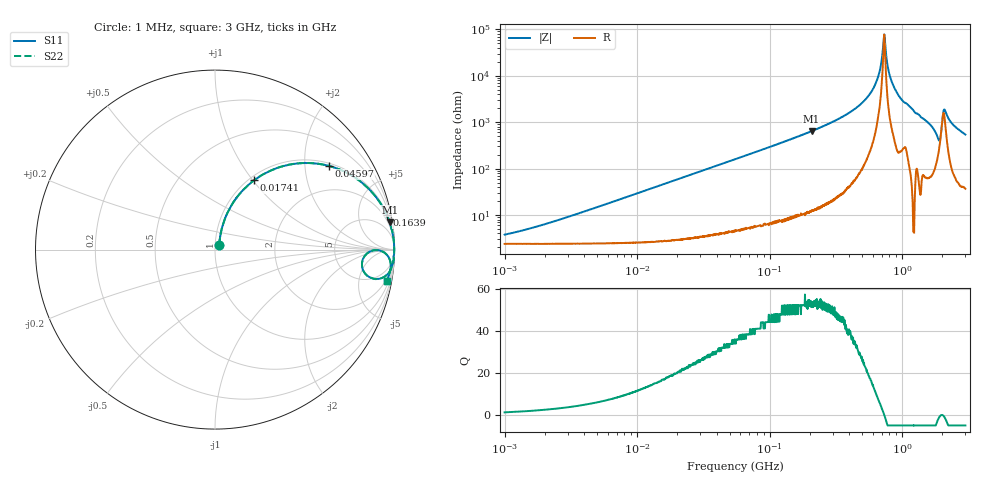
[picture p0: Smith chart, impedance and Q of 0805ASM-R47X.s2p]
!s-Parameter Generated by FASTRON Sdn. Bhd.
!FASTRON P/N : 0805ASM-R47X
!Keysight Technologies: E4991B_MY54100416_A.01.15
!Date: Fri Jun 19 14:52:53 2026
!Version  :Rev00  Fri Jun 19 14:52:53 2026
!Data & Calibration Information:
!Freq  S11  S21  S12  S22
!PortZ  Port1:50+j0  Port2:50+j0
!When reading reference impedance value at option line is always used.
! Remarks : This data is being provided solely for informational purposes.
# Hz S dB R 50
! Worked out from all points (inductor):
!   1601 points, 1 MHz to 3 GHz, reference 50 ohm
!   read as one part in series: L = 465 nH near 2.474 MHz
!   highest Q = 54 at 207.3 MHz (marker M1), where L = 494 nH
!   self-resonance near 731.6 MHz
!   S11 on the Smith chart (normalised r, x): 1 MHz: 1.05, +0.06; 17.41 MHz: 1.06, +1.01; 45.97 MHz: 1.08, +2.67; 163.9 MHz: 1.20, +9.87; 3 GHz: 2, -11
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1000000  -28.70 49.1  -0.21 -1.6  -0.21 -1.6  -28.70 49.1
3804036  -19.10 71.5  -0.26 -6.2  -0.26 -6.2  -19.10 71.5
1.447069e7  -8.39 64.0  -0.91 -22.3  -0.91 -22.3  -8.39 64.0
1.741396e7  -7.07 60.6  -1.19 -26.3  -1.19 -26.3  -7.07 60.6
4.597255e7  -2.06 36.2  -4.57 -52.0  -4.57 -52.0  -2.06 36.2
5.504702e7  -1.55 31.6  -5.62 -56.8  -5.62 -56.8  -1.55 31.6
1.63867e8  -0.21 11.4  -14.00 -77.4  -14.00 -77.4  -0.21 11.4
2.073156e8  -0.13 8.8  -16.30 -80.1  -16.30 -80.1  -0.13 8.8
2.083556e8  -0.13 8.8  -16.30 -80.1  -16.30 -80.1  -0.13 8.8
3.760477e8  -0.04 4.0  -23.20 -84.7  -23.20 -84.7  -0.04 4.0
5.391547e8  -0.02 1.7  -30.40 -85.5  -30.40 -85.5  -0.02 1.7
6.488164e8  -0.01 0.7  -38.40 -82.7  -38.40 -82.7  -0.01 0.7
7.279565e8  -0.01 0.0  -56.90 -25.1  -56.90 -25.1  -0.01 0.0
7.50144e8  -0.01 -0.1  -51.40 63.2  -51.40 63.2  -0.01 -0.1
7.925923e8  -0.01 -0.5  -41.70 81.3  -41.70 81.3  -0.01 -0.5
8.543737e8  -0.01 -0.9  -36.00 84.1  -36.00 84.1  -0.01 -0.9
9.682285e8  -0.02 -1.7  -30.50 84.3  -30.50 84.3  -0.02 -1.7
1.855641e9  -0.81 -10.4  -14.20 57.6  -14.20 57.6  -0.81 -10.4
1.921792e9  -1.67 -6.7  -13.80 28.0  -13.80 28.0  -1.67 -6.7
2.102926e9  -0.28 -2.5  -25.40 52.5  -25.40 52.5  -0.28 -2.5
2.41921e9  -0.14 -6.3  -19.10 78.5  -19.10 78.5  -0.14 -6.3
3e9  -0.25 -10.3  -14.90 75.8  -14.90 75.8  -0.25 -10.3
